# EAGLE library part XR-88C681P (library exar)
DUAL UART full duplex
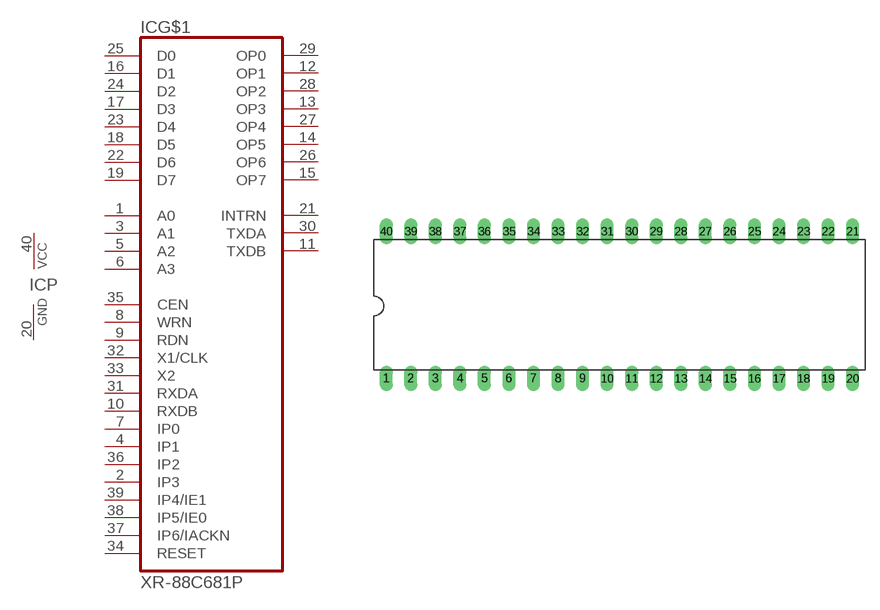
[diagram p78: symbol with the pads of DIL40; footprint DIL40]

Designator prefix IC; gates G$1=88C681P P=PWRN

## XR-88C681P (MPN: XR88C681CP/40-F; OC_FARNELL: 1095818; OC_NEWARK: 53R0425)  [DIL40]
1  G$1:A0  in
2  G$1:IP3  in
3  G$1:A1  in
4  G$1:IP1  in
5  G$1:A2  in
6  G$1:A3  in
7  G$1:IP0  in
8  G$1:WRN  in
9  G$1:RDN  in
10  G$1:RXDB  in
11  G$1:TXDB  out
12  G$1:OP1  out
13  G$1:OP3  out
14  G$1:OP5  out
15  G$1:OP7  out
16  G$1:D1
17  G$1:D3
18  G$1:D5
19  G$1:D7
20  P:GND  pwr
21  G$1:INTRN  out
22  G$1:D6
23  G$1:D4
24  G$1:D2
25  G$1:D0
26  G$1:OP6  out
27  G$1:OP4  out
28  G$1:OP2  out
29  G$1:OP0  out
30  G$1:TXDA  out
31  G$1:RXDA  in
32  G$1:X1/CLK  in
33  G$1:X2  in
34  G$1:RESET  in
35  G$1:CEN  in
36  G$1:IP2  in
37  G$1:IP6/IACKN  in
38  G$1:IP5/IE0
39  G$1:IP4/IE1  in
40  P:VCC  pwr

## Footprint DIL40 (pad centres in mm)
Dual In Line Package
drill 0.813 long: 1 -24.13,-7.62; 2 -21.59,-7.62; 3 -19.05,-7.62; 4 -16.51,-7.62; 5 -13.97,-7.62; 6 -11.43,-7.62; 7 -8.89,-7.62; 8 -6.35,-7.62; 9 -3.81,-7.62; 10 -1.27,-7.62; 11 1.27,-7.62; 12 3.81,-7.62; 13 6.35,-7.62; 14 8.89,-7.62; 15 11.43,-7.62; 16 13.97,-7.62; 17 16.51,-7.62; 18 19.05,-7.62; 19 21.59,-7.62; 20 24.13,-7.62; 21 24.13,7.62; 22 21.59,7.62; 23 19.05,7.62; 24 16.51,7.62; 25 13.97,7.62; 26 11.43,7.62; 27 8.89,7.62; 28 6.35,7.62; 29 3.81,7.62; 30 1.27,7.62; 31 -1.27,7.62; 32 -3.81,7.62; 33 -6.35,7.62; 34 -8.89,7.62; 35 -11.43,7.62; 36 -13.97,7.62; 37 -16.51,7.62; 38 -19.05,7.62; 39 -21.59,7.62; 40 -24.13,7.62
